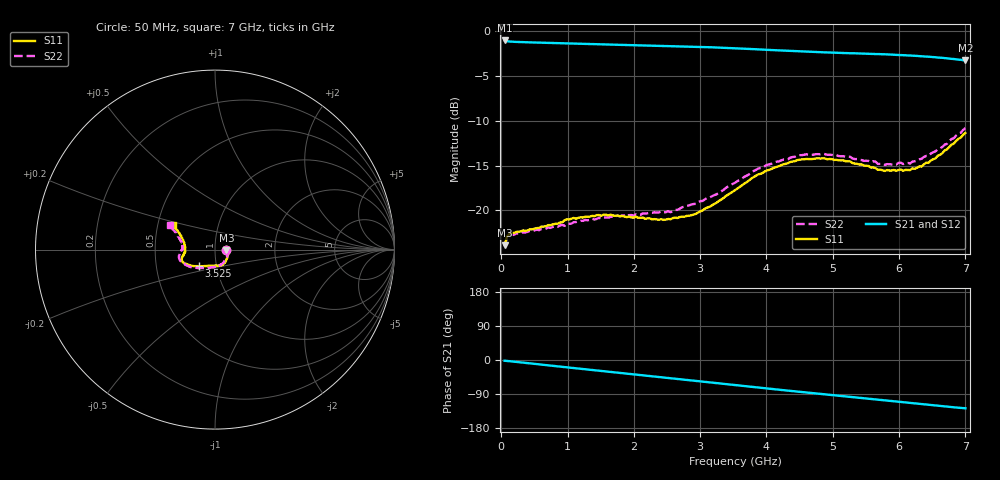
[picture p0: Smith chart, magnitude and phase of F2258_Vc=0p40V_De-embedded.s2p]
! Integrated Device Technology
! Corporate Headquarters
! 6024 Silver Creek Valley Road
! San Jose, CA 95138  USA
! Phone:  1-408-284-8200
! Toll Free:  1-800-223-1366
! Webpage:  http://www.idt.com/
! Timing and RF Division
! 515 Groton Road, Suite 102
! Westford, MA 01886-6024
! Device:  F2258
! Description: Voltage Variable RF Attenuator
! Frequency:  50.0 -  6000.00 MHz
! Package:  3x3 mm Thin QFN Plastic Package: 16 pin
! Ports:  2 RF, 2 DC
!  Pin  1  = NC
!  Pin  2  = NC
!  Pin  3  = RF2  = Port 2
!  Pin  4  = GND
!  Pin  5  = Vdd
!  Pin  6  = NC
!  Pin  7  = VCTRL
!  Pin  8  = NC
!  Pin  9  = GND
!  Pin 10  = RF1  = Port 1
!  Pin 11  = NC
!  Pin 12  = NC
!  Pin 13  = NC
!  Pin 14  = NC
!  Pin 15  = NC
!  Pin 16  = NC
! Vcntrl:  0.400 Volts
! Vdd:  +3.300 Volts
! Current:  1.093 mA
! Data:  The device was measured on a the F2258 evaluation board which has
!  individual transmission lines to the RF pins.  Data was collected
!  using a calibrated network analyzer.  The evaluation board was
!  de-embedded using a TRL calibration technique.
!  The reference plane is the edge of the package pin.
! Misc:  SN 10
!  Action Tracker AT0285
! Date Measured:  2014-12-10
! Date:  2016-01-13  MJV
! Note:
!  Integrated Device Technology supplies this data as a sample of measured
!  data at the package pin for this product.  Your particular data for this
!  product may vary.
!  Data was taken at 25 degrees C.
!  Integrated Device Technology reserves the right to change this data at anytime.
!Freq_(GHz)  S11M_(dB)  S11P_(deg)  S21M_(dB)  S21P_(deg)  S12M_(dB)  S12P_(deg)  S22M_(dB)  S22P_(deg)
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# GHz S dB R 50
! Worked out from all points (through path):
!   201 points, 50 MHz to 7 GHz, reference 50 ohm
!   highest |S21| = -1.02 dB at 50 MHz (marker M1); lowest = -3.3 dB at 7 GHz (marker M2)
!   group delay of S21, straight-line fit = 50.5 ps
!   lowest |S11| = -23.9 dB at 50 MHz (marker M3), VSWR 1.14, Z = 56.8 - j0.417 ohm
!   |S11| at or under -10 dB: start of sweep to end of sweep
!   |S22| runs from -24.0 to -10.8 dB; largest |S21 - S12| = 0.00048
!   S11 on the Smith chart (normalised r, x): 50 MHz: 1.14, -0.01; 3.525 GHz: 0.82, -0.15; 7 GHz: 0.60, +0.18
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0.05  -23.91 -3.3  -1.02 -2.0  -1.02 -1.9  -24.01 -3.1
0.08475  -22.97 -5.4  -1.10 -2.5  -1.10 -2.5  -23.09 -5.2
0.15425  -22.51 -8.5  -1.16 -3.6  -1.16 -3.6  -22.73 -9.0
0.71025  -21.65 -34.6  -1.29 -14.1  -1.29 -14.1  -21.93 -37.1
0.98825  -21.01 -47.9  -1.34 -19.4  -1.34 -19.4  -21.51 -52.6
1.2315  -20.81 -55.9  -1.40 -23.8  -1.40 -23.8  -21.17 -61.6
1.6485  -20.49 -67.4  -1.48 -31.4  -1.48 -31.4  -20.73 -74.7
2.37825  -21.06 -87.8  -1.61 -44.8  -1.61 -44.8  -20.23 -92.7
2.552  -21.00 -93.7  -1.65 -48.0  -1.64 -48.0  -20.20 -98.0
2.93425  -20.40 -110.5  -1.73 -55.1  -1.73 -55.1  -19.28 -111.5
3.247  -19.16 -123.5  -1.80 -61.0  -1.80 -61.0  -18.22 -123.8
3.525  -17.76 -134.4  -1.89 -66.2  -1.89 -66.2  -16.92 -134.4
4.0115  -15.54 -148.8  -2.07 -75.2  -2.07 -75.2  -14.91 -150.0
4.46325  -14.40 -157.6  -2.23 -83.4  -2.23 -83.4  -13.89 -161.3
4.7065  -14.26 -160.9  -2.30 -87.7  -2.30 -87.7  -13.79 -165.6
5.2625  -14.54 -167.7  -2.45 -97.4  -2.46 -97.4  -14.02 -173.7
5.6795  -15.48 -174.3  -2.54 -104.6  -2.54 -104.6  -14.82 -179.3
5.85325  -15.55 -178.4  -2.59 -107.8  -2.60 -107.8  -14.85 176.1
6.166  -15.51 173.6  -2.70 -113.4  -2.70 -113.4  -14.77 170.1
6.33975  -15.11 167.1  -2.78 -116.5  -2.78 -116.5  -14.25 165.7
6.722  -13.20 154.9  -3.01 -123.1  -3.02 -123.1  -12.58 156.6
7  -11.36 149.2  -3.26 -127.4  -3.26 -127.4  -10.82 151.6
